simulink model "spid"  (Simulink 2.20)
settings: Solver=ode4  StartTime=0.0  StopTime=100  FixedStep=2  RelTol=1e-3  AbsTol=1e-6
libraries: simulink x1

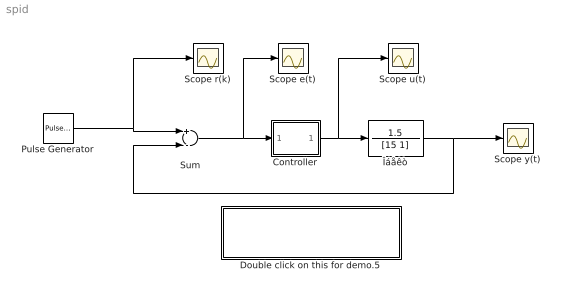
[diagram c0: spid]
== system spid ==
  Controller : Subsystem  mask(Controller){P=0.1, I=1.5, D=2}
      mask prompts: P "Proportional :"; I "Integral :"; D "Derivative :"
      mask help: Enter expressions for proportional, integral, and derivative terms.
      mask init:
      | P=@1; I=@2; D=@3;
  Double click on this for demo.5 : Subsystem
  Pulse Generator : simulink/Sources/Pulse Generator  period=250  duty=50  amplitude=1  start=0
  Scope e(t) : Scope
  Scope r(k) : Scope
  Scope u(t) : Scope
  Scope y(t) : Scope
  Sum : Sum  Inputs=+-
  Îáåêò : TransferFcn  Numerator=1.5  Denominator=[15 1]
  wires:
  Controller/1(Out_1) -> Îáåêò/1, Scope u(t)/1
  Pulse Generator/1 -> Sum/1, Scope r(k)/1
  Îáåêò/1 -> Scope y(t)/1, Sum/2
  Sum/1 -> Controller/1(In_1), Scope e(t)/1

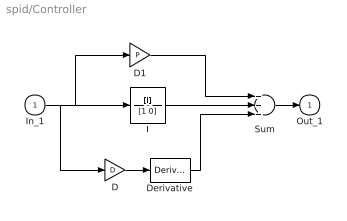
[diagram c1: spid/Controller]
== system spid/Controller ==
  In_1 : Inport  Port=1  PortWidth=-1  SampleTime=-1
  D : Gain  Gain=D
  D1 : Gain  Gain=P
  Derivative : Derivative
  I : TransferFcn  Numerator=[I]  Denominator=[1 0]
  Sum : Sum  Inputs=+++
  Out_1 : Outport  Port=1  InitialOutput=0
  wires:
  In_1/1 -> D1/1, I/1, D/1
  Sum/1 -> Out_1/1
  D/1 -> Derivative/1
  Derivative/1 -> Sum/3
  I/1 -> Sum/2
  D1/1 -> Sum/1

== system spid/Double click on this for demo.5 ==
